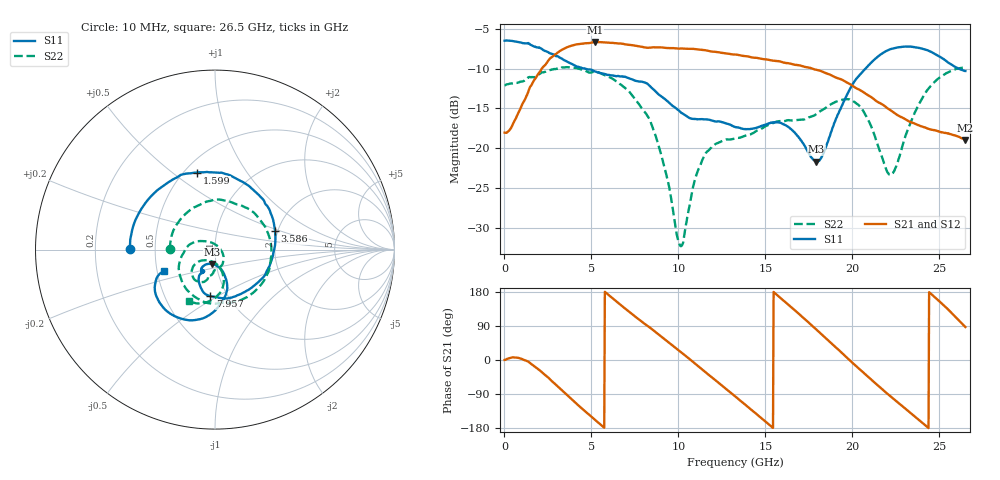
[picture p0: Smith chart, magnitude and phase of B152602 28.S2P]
!  2-Port S-parameters saved by WinCal
! VAR MeasName=S-Parameters (CALIBRATED_DATA) read from VNA (N5242A)
! VAR MeasDate=2016-1-5 16:30:17
! VAR NAME=B152602 28
! VAR FILENAME=B152602 28.S2P
! VAR DATE=2016-1-5 16:30:17
! VAR PHYS_PORTS=1,2
# Hz S DB R 50
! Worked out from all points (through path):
!   801 points, 10 MHz to 26.5 GHz, reference 50 ohm
!   highest |S21| = -6.66 dB at 5.209 GHz (marker M1); lowest = -19.0 dB at 26.5 GHz (marker M2)
!   lowest |S11| = -21.7 dB at 17.92 GHz (marker M3), VSWR 1.18, Z = 47.7 - j7.71 ohm
!   |S11| at or under -10 dB: 4.631 GHz to 20.76 GHz (16.13 GHz wide, 127 % of centre); 26.11 GHz to end of sweep
!   |S22| runs from -32.3 to -9.8 dB; largest |S21 - S12| = 0.0028
!   S11 on the Smith chart (normalised r, x): 10 MHz: 0.36, +0.00; 1.599 GHz: 0.58, +0.61; 3.586 GHz: 1.94, +0.45; 7.957 GHz: 0.83, -0.46; 26.5 GHz: 0.55, -0.14
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1e7  -6.49 179.5  -18.06 0.2  -18.05 -0.1  -12.10 179.5
1.5994e9  -7.11 103.2  -11.85 -12.3  -11.85 -12.3  -11.07 74.9
2.592775e9  -8.04 58.2  -8.79 -49.8  -8.79 -49.8  -10.20 16.8
3.58615e9  -9.11 17.0  -7.32 -91.9  -7.33 -91.9  -9.82 -33.2
4.447075e9  -9.92 -11.9  -6.87 -127.9  -6.87 -127.8  -10.14 -68.7
5.208662e9  -10.35 -34.8  -6.66 -157.9  -6.65 -157.8  -10.40 -92.9
6.400712e9  -10.96 -63.3  -6.81 155.9  -6.79 156.0  -11.55 -130.4
7.957e9  -11.68 -95.9  -7.28 99.0  -7.28 99.1  -15.17 -174.8
8.851038e9  -13.22 -112.3  -7.32 67.9  -7.29 67.8  -19.59 153.3
1.014242e10  -15.52 -121.3  -7.46 21.0  -7.44 20.9  -32.35 44.7
1.146692e10  -16.37 -119.6  -7.67 -28.7  -7.65 -28.8  -21.07 -60.9
1.3255e10  -17.34 -122.3  -8.24 -95.5  -8.23 -95.7  -18.79 -91.1
1.441394e10  -17.49 -117.1  -8.63 -139.6  -8.62 -139.8  -17.95 -93.9
1.544042e10  -16.78 -118.3  -9.00 -179.2  -8.96 -179.3  -16.86 -98.3
1.666559e10  -18.00 -126.1  -9.51 132.3  -9.46 132.2  -16.53 -104.5
1.769208e10  -21.28 -112.6  -9.99 90.1  -9.97 90.2  -16.00 -103.8
1.792386e10  -21.70 -102.2  -10.15 80.7  -10.12 80.5  -15.74 -104.0
1.918214e10  -15.70 -69.3  -11.23 27.9  -11.20 27.9  -14.08 -113.7
2.030796e10  -11.08 -80.2  -12.55 -19.6  -12.50 -19.7  -14.49 -133.1
2.209604e10  -7.64 -108.3  -15.11 -92.2  -15.03 -92.5  -23.29 -117.1
2.431458e10  -7.69 -143.4  -17.52 -177.2  -17.52 -177.4  -12.69 -81.1
2.65e10  -10.30 -157.3  -18.97 87.0  -18.96 86.7  -9.83 -116.5
